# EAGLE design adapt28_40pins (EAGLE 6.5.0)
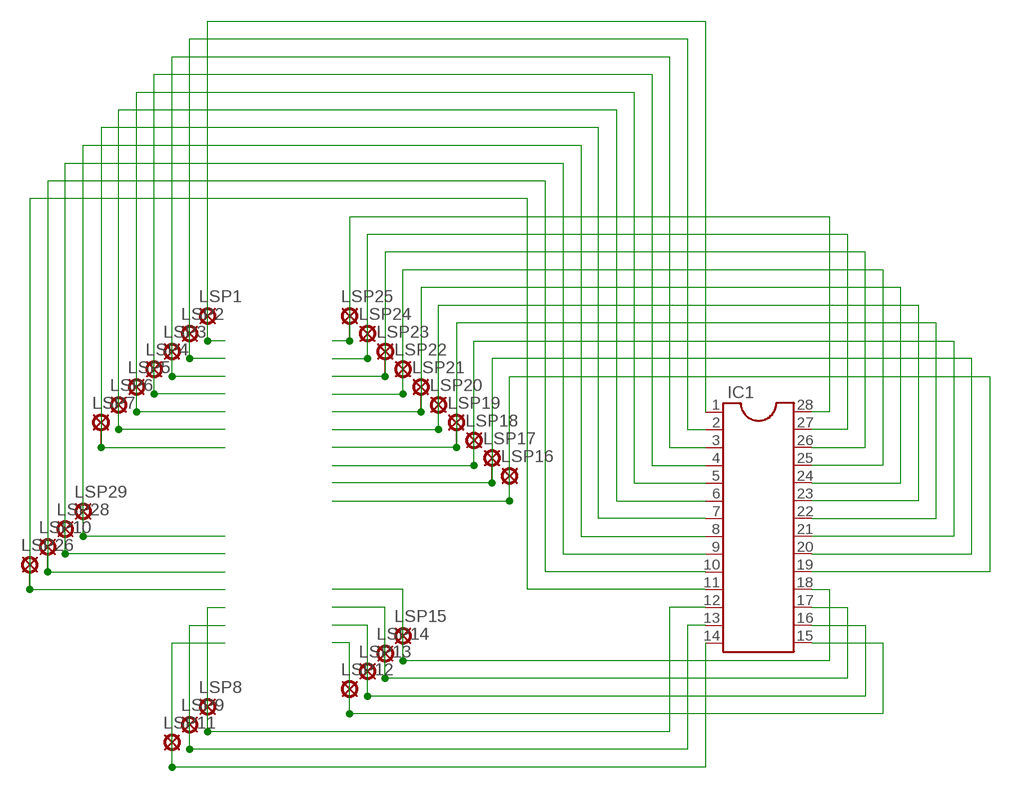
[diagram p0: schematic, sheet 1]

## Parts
IC1  DIL28-3  [DIL28-3]
LSP1  LSP10  [LSP10]
LSP2  LSP10  [LSP10]
LSP3  LSP10  [LSP10]
LSP4  LSP10  [LSP10]
LSP5  LSP10  [LSP10]
LSP6  LSP10  [LSP10]
LSP7  LSP10  [LSP10]
LSP8  LSP10  [LSP10]
LSP9  LSP10  [LSP10]
LSP10  LSP10  [LSP10]
LSP11  LSP10  [LSP10]
LSP12  LSP10  [LSP10]
LSP13  LSP10  [LSP10]
LSP14  LSP10  [LSP10]
LSP15  LSP10  [LSP10]
LSP16  LSP10  [LSP10]
LSP17  LSP10  [LSP10]
LSP18  LSP10  [LSP10]
LSP19  LSP10  [LSP10]
LSP20  LSP10  [LSP10]
LSP21  LSP10  [LSP10]
LSP22  LSP10  [LSP10]
LSP23  LSP10  [LSP10]
LSP24  LSP10  [LSP10]
LSP25  LSP10  [LSP10]
LSP26  LSP10  [LSP10]
LSP28  LSP10  [LSP10]
LSP29  LSP10  [LSP10]

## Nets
N$1: IC1.1 LSP1.MP
N$2: IC1.2 LSP2.MP
N$3: IC1.3 LSP3.MP
N$4: IC1.4 LSP4.MP
N$5: IC1.5 LSP5.MP
N$6: IC1.6 LSP6.MP
N$7: IC1.7 LSP7.MP
N$8: IC1.8 LSP29.MP
N$9: IC1.9 LSP28.MP
N$10: IC1.10 LSP10.MP
N$11: IC1.11 LSP26.MP
N$12: IC1.28 LSP25.MP
N$13: IC1.27 LSP24.MP
N$14: IC1.26 LSP23.MP
N$15: IC1.25 LSP22.MP
N$16: IC1.24 LSP21.MP
N$17: IC1.23 LSP20.MP
N$18: IC1.22 LSP19.MP
N$19: IC1.21 LSP18.MP
N$20: IC1.20 LSP17.MP
N$21: IC1.19 LSP16.MP
N$22: IC1.14 LSP11.MP
N$23: IC1.13 LSP9.MP
N$24: IC1.12 LSP8.MP
N$25: IC1.15 LSP12.MP
N$26: IC1.16 LSP13.MP
N$27: IC1.17 LSP14.MP
N$28: IC1.18 LSP15.MP

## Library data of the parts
IC1 = ic-package:DIL28: Dual In Line
LSP1-LSP26 LSP28 LSP29 = solpad:LSP10: SOLDER PAD

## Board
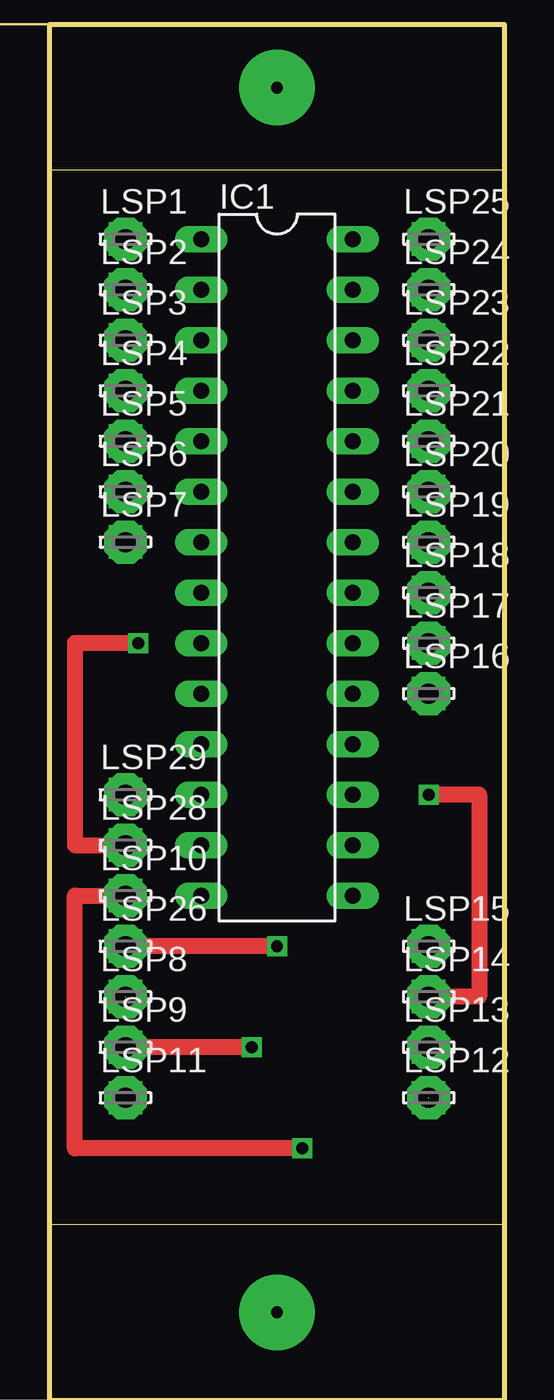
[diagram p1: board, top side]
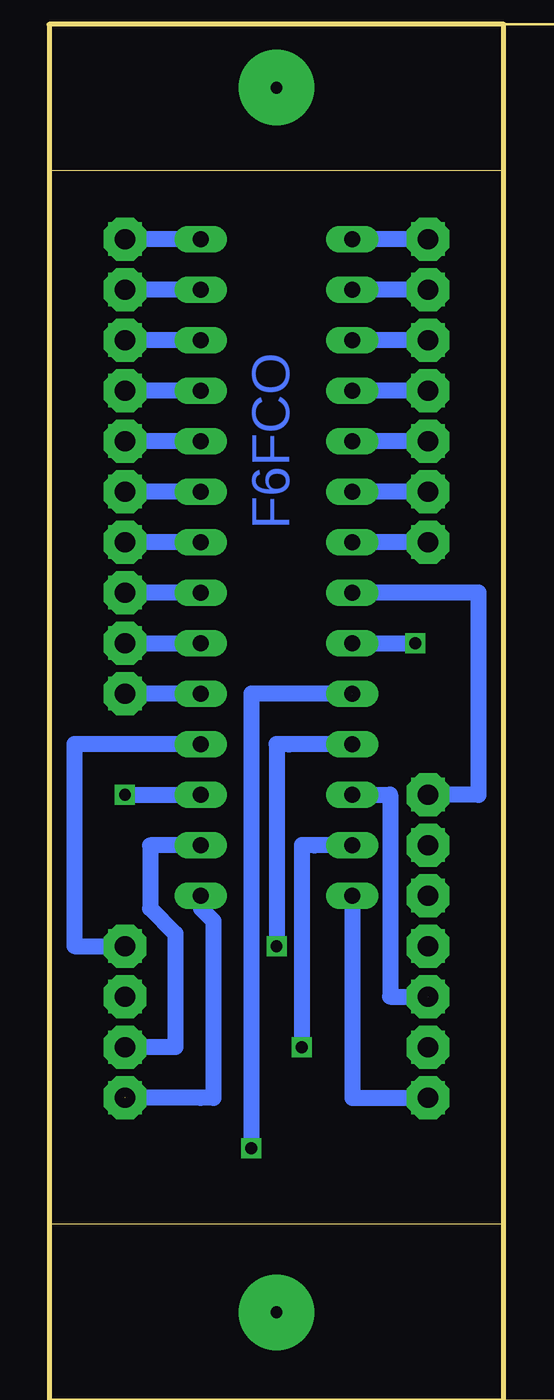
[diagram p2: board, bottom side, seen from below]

Size 22.84 x 53.01 mm. Coordinates in mm from the lower left corner, seen from the top.
Outline: 0,0 22.84,0 22.84,53.01 0,53.01 0,0
Copper layers (1*16): Top 0.035mm / dielectric 1.5mm / Bottom 0.035mm
Design rules "default": minimum track width 10mil, minimum drill 24mil, track to track 8mil, track to pad 8mil, pad to pad 8mil, via to via 8mil, smd to smd 8mil, copper to edge 40mil, drill to drill 8mil, minimum pad ring 10mil, minimum via ring 8mil, stop-mask expansion 4mil, vias tented up to drill 0mil, thermal gap 10mil
Milling: area -13,58.8 to -12.4,60.3; area -13,-8.9 to -12.4,-7.4; area -12.3,22.3 to -10.5,29.2; 7 lines

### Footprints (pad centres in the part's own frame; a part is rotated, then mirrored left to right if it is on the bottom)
DIL28-3 = drill 0.813 long: 1 -16.51,-3.81; 2 -13.97,-3.81; 3 -11.43,-3.81; 4 -8.89,-3.81; 5 -6.35,-3.81; 6 -3.81,-3.81; 7 -1.27,-3.81; 8 1.27,-3.81; 9 3.81,-3.81; 10 6.35,-3.81; 11 8.89,-3.81; 12 11.43,-3.81; 13 13.97,-3.81; 14 16.51,-3.81; 15 16.51,3.81; 16 13.97,3.81; 17 11.43,3.81; 18 8.89,3.81; 19 6.35,3.81; 20 3.81,3.81; 21 1.27,3.81; 22 -1.27,3.81; 23 -3.81,3.81; 24 -6.35,3.81; 25 -8.89,3.81; 26 -11.43,3.81; 27 -13.97,3.81; 28 -16.51,3.81
LSP10 = drill 1.016 pad 2.159 octagon: MP 0,0

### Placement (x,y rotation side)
IC1  11.43,33.02 270 top
LSP1  3.81,49.54 0 top
LSP2  3.81,47 0 top
LSP3  3.81,44.46 0 top
LSP4  3.81,41.92 0 top
LSP5  3.81,39.38 0 top
LSP6  3.81,36.84 0 top
LSP7  3.81,34.3 0 top
LSP8  3.81,11.43 0 top
LSP9  3.81,8.89 0 top
LSP10  3.81,16.51 0 top
LSP11  3.81,6.35 0 top
LSP12  19.05,6.35 0 top
LSP13  19.05,8.89 0 top
LSP14  19.05,11.43 0 top
LSP15  19.05,13.97 0 top
LSP16  19.05,26.68 0 top
LSP17  19.05,29.22 0 top
LSP18  19.05,31.76 0 top
LSP19  19.05,34.3 0 top
LSP20  19.05,36.84 0 top
LSP21  19.05,39.38 0 top
LSP22  19.05,41.92 0 top
LSP23  19.05,44.46 0 top
LSP24  19.05,47 0 top
LSP25  19.05,49.54 0 top
LSP26  3.81,13.97 0 top
LSP28  3.81,19.05 0 top
LSP29  3.81,21.59 0 top

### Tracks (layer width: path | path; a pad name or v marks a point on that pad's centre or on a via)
N$1
  Bottom 0.813: LSP1.MP IC1.1
N$2
  Bottom 0.813: LSP2.MP IC1.2
N$3
  Bottom 0.813: LSP3.MP IC1.3
N$4
  Bottom 0.813: LSP4.MP IC1.4
N$5
  Bottom 0.813: LSP5.MP IC1.5
N$6
  Bottom 0.813: LSP6.MP IC1.6
N$7
  Bottom 0.813: LSP7.MP IC1.7
N$8
  Bottom 0.813: IC1.8 1.27,31.76 1.27,21.59 1.28,21.59 LSP29.MP
N$9  (via drill 0.6 pad 0.81)
  Top 0.813: v4.45,29.22 1.27,29.22 1.27,19.05 LSP28.MP
  Bottom 0.813: IC1.9 v4.45,29.21 v4.45,29.22
N$10  (via drill 0.6 pad 0.81)  (1 unrouted)
  Top 0.813: v12.7,3.81 1.27,3.81 1.27,16.51 LSP10.MP
  Bottom 0.813: IC1.10 12.7,26.67 v12.7,3.81
N$11  (via drill 0.6 pad 0.81)
  Top 0.813: v11.43,13.97 LSP26.MP
  Bottom 0.813: IC1.11 10.79,24.13 11.43,24.13 v11.43,13.97
N$12
  Bottom 0.813: IC1.28 LSP25.MP
N$13
  Bottom 0.813: IC1.27 LSP24.MP
N$14
  Bottom 0.813: IC1.26 LSP23.MP
N$15
  Bottom 0.813: IC1.25 LSP22.MP
N$16
  Bottom 0.813: IC1.24 LSP21.MP
N$17
  Bottom 0.813: IC1.23 LSP20.MP
N$18
  Bottom 0.813: IC1.22 LSP19.MP
N$19
  Bottom 0.813: IC1.21 LSP18.MP
N$20
  Bottom 0.813: LSP17.MP IC1.20
N$21
  Bottom 0.813: IC1.19 LSP16.MP
N$22
  Bottom 0.813: IC1.14 7.62,6.35 LSP11.MP
N$23  (via drill 0.6 pad 0.81)
  Top 0.813: v10.16,8.89 LSP9.MP
  Bottom 0.813: IC1.13 9.52,19.05 10.16,19.05 v10.16,8.89
N$24  (1 unrouted)
  Bottom 0.813: IC1.12 5.72,21.59 5.72,11.43 LSP8.MP
N$25  (1 unrouted)
  Bottom 0.813: 15.24,6.36 15.24,6.35 | 15.24,6.35 LSP12.MP | IC1.15 15.24,15.87 14.61,15.24 14.61,6.35 15.24,6.35
N$26
  Bottom 0.813: IC1.16 17.78,19.05 17.78,15.88 16.51,14.61 16.51,8.89 LSP13.MP
N$27  (via drill 0.6 pad 0.81)
  Top 0.813: LSP14.MP 21.59,11.43 21.59,21.59 v19.06,21.59 v19.05,21.59
  Bottom 0.813: v19.05,21.59 IC1.17
N$28
  Bottom 0.813: IC1.18 21.59,24.13 21.59,13.97 LSP15.MP
N$29  (via drill 0.6 pad 1.68)
  other vias: 3.81,49.55
N$30  (via drill 0.6 pad 1.68)
  other vias: 3.81,47.01
N$31  (via drill 0.6 pad 1.68)
  other vias: 3.81,44.47
N$32  (via drill 0.6 pad 1.68)
  other vias: 3.81,41.93
N$33  (via drill 0.6 pad 1.68)
  other vias: 3.81,39.39
N$34  (via drill 0.6 pad 1.68)
  other vias: 3.81,36.85
N$35  (via drill 0.6 pad 1.68)
  other vias: 3.81,34.31
N$36  (via drill 0.6 pad 1.68)
  other vias: 3.81,21.6
N$37  (via drill 0.6 pad 1.68)
  other vias: 3.81,19.06
N$38  (via drill 0.6 pad 1.68)
  other vias: 3.81,16.52
N$39  (via drill 0.6 pad 1.68)
  other vias: 3.81,13.98
N$40  (via drill 0.6 pad 1.68)
  other vias: 3.81,11.44
N$41  (via drill 0.6 pad 1.68)
  other vias: 3.81,8.9
N$42  (via drill 0.6 pad 1.68)
  other vias: 3.81,6.36
N$47  (via drill 0.6 pad 1.68)
  other vias: 19.06,6.36
N$48  (via drill 0.6 pad 1.68)
  other vias: 19.06,8.9
N$49  (via drill 0.6 pad 1.68)
  other vias: 19.06,11.44
N$50  (via drill 0.6 pad 1.68)
  other vias: 19.06,13.98
N$51  (via drill 0.6 pad 1.68)
  other vias: 19.06,26.68
N$52  (via drill 0.6 pad 1.68)
  other vias: 19.06,29.22
N$53  (via drill 0.6 pad 1.68)
  other vias: 19.06,31.77
N$54  (via drill 0.6 pad 1.68)
  other vias: 19.06,34.31
N$55  (via drill 0.6 pad 1.68)
  other vias: 19.06,36.85
N$56  (via drill 0.6 pad 1.68)
  other vias: 19.06,39.39
N$57  (via drill 0.6 pad 1.68)
  other vias: 19.06,41.93
N$58  (via drill 0.6 pad 1.68)
  other vias: 19.06,44.47
N$59  (via drill 0.6 pad 1.68)
  other vias: 19.06,47.01
N$60  (via drill 0.6 pad 1.68)
  other vias: 19.06,49.55
N$61  (via drill 0.6 pad 3.81)
  other vias: 11.43,57.16
N$62  (via drill 0.6 pad 3.81)
  other vias: 11.43,-4.44

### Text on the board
Bottom: F6FCO
Vias: Centrage CNC | Centrage CNC
Document: Adaptateur PIC / 28pins > 40pins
